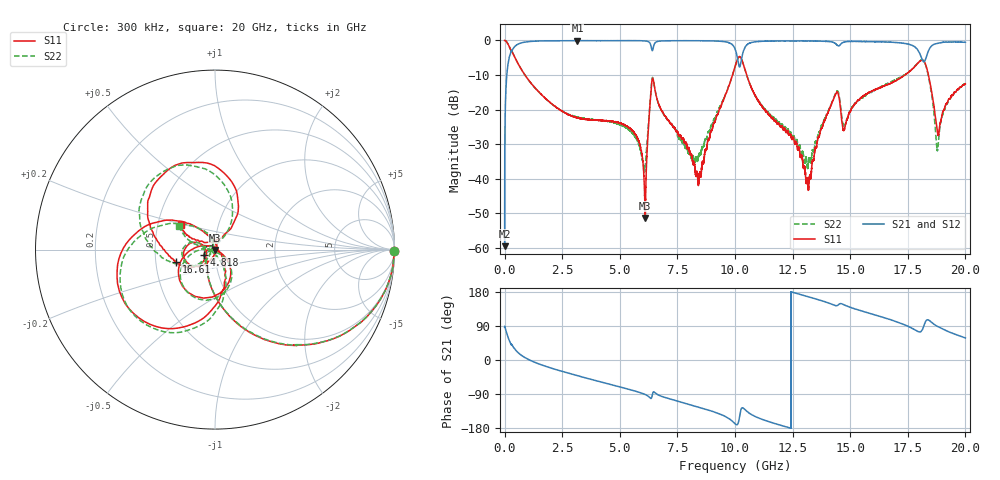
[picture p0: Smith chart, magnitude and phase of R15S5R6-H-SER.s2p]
!{R15S5R6}
!Johanson Technology Inc.
!www.johansontechnology.com
!Test Board Conditions:
!Substrate Type  RO4350B
!Substrate Thickness  20 mil
!Substrate Dk  3.66
!TL Type: GCPW
!TL Trace Width  34 mil
!TL Gap  10 mil
!Electrode orientation  Horizontal
!DUT TOPOLOGY	SERIES
!Mounting Pad LxW  26x52 mil
! Created Sat Feb  6 13:59:08 2021
# hz S ma R 50
! 2 Port Network Data from SP1.SP block
! freq  magS11  angS11  magS21  angS21  magS12  angS12  magS22  angS22
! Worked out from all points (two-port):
!   20001 points, 300 kHz to 20 GHz, reference 50 ohm
!   highest |S21| = -0.04 dB at 3.159 GHz (marker M1); lowest = -59.6 dB at 300 kHz (marker M2)
!   |S21| within 3 dB of the highest: 311.6 MHz to 10.03 GHz (9.723 GHz wide, 188 % of centre); 10.37 GHz to 17.96 GHz (7.594 GHz wide, 53.6 % of centre)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
!   lowest |S11| = -51.4 dB at 6.104 GHz (marker M3), VSWR 1.01, Z = 50 - j0.267 ohm
!   |S11| at or under -10 dB: 883.1 MHz to 9.896 GHz (9.012 GHz wide, 167 % of centre); 10.51 GHz to 17.38 GHz (6.872 GHz wide, 49.3 % of centre); 18.4 GHz to end of sweep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
!   |S22| runs from -38.1 to 0.0 dB; largest |S21 - S12| = 0.016
!   S11 on the Smith chart (normalised r, x): 300 kHz: open; 4.818 GHz: 0.88, -0.05; 16.61 GHz: 0.64, -0.09; 20 GHz: 0.65, +0.19
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300000  1 -0.4  0.001052 86.3  0.001043 86.4  0.999 -0.3
1.133e8  0.9292 -23.2  0.3653 66.6  0.3661 66.6  0.9289 -23.1
3.203e8  0.6947 -50.2  0.7146 39.6  0.7157 39.6  0.6947 -50.0
1.0973e9  0.2527 -90.3  0.9654 -0.4  0.9654 -0.5  0.252 -90.2
3.1593e9  0.07553 -127.7  0.995 -41.3  0.9934 -41.4  0.07702 -132.9
3.3343e9  0.07409 -129.8  0.9933 -44.2  0.9927 -44.3  0.07561 -135.6
4.8183e9  0.06649 -155.2  0.993 -68.1  0.992 -68.1  0.06436 -157.8
5.7343e9  0.04099 -177.8  0.9931 -83.3  0.993 -83.3  0.037 -163.5
6.1043e9  0.002686 -94.9  0.984 -91.2  0.9858 -91.1  0.01554 -76.1
6.3893e9  0.2543 -87.9  0.7368 -98.3  0.7365 -98.1  0.2645 -85.5
6.6673e9  0.1247 178.4  0.9722 -92.1  0.973 -92.0  0.1246 -171.1
8.4423e9  0.01035 35.9  0.99 -124.7  0.9893 -124.7  0.02179 -105.7
1.00003e10  0.4145 -103.8  0.7571 -168.1  0.7577 -167.9  0.4149 -98.3
1.05333e10  0.2981 146.3  0.8715 -136.3  0.8727 -136.5  0.2963 151.0
1.33343e10  0.01515 -79.6  0.9823 164.2  0.9823 164.2  0.02256 -161.3
1.43813e10  0.17 -153.9  0.8917 143.3  0.8915 143.2  0.1775 -155.0
1.47393e10  0.05045 -158.8  0.9466 145.4  0.9506 145.4  0.05756 -165.5
1.66083e10  0.2274 -162.3  0.9469 109.1  0.9441 108.9  0.2371 -160.9
1.66673e10  0.2339 -165.0  0.9491 107.8  0.937 107.6  0.2421 -162.0
1.81833e10  0.5008 104.4  0.4906 87.3  0.4901 88.0  0.5125 114.2
1.87923e10  0.04624 93.8  0.9065 88.6  0.9055 88.7  0.02612 124.0
2e10  0.237 144.3  0.9397 58.1  0.9321 57.7  0.2388 146.4
